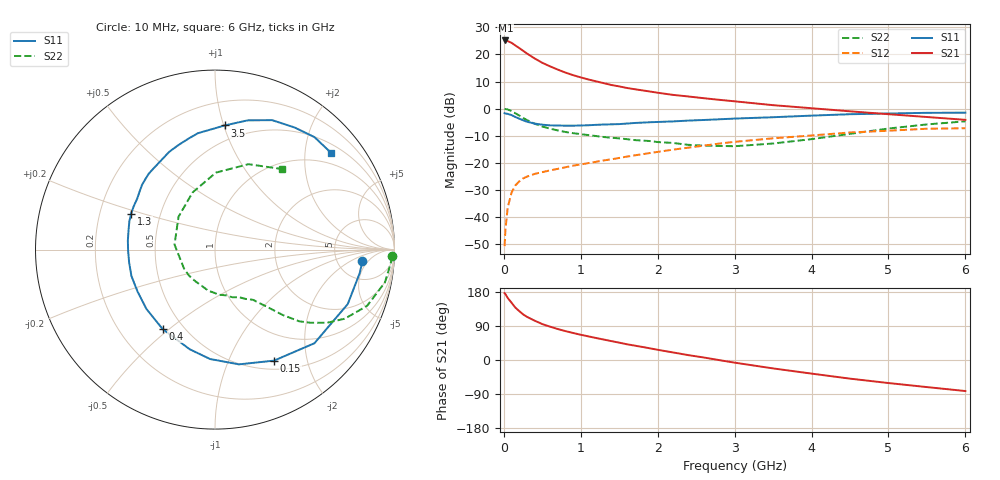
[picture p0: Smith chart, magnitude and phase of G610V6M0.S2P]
! SIEMENS Small Signal Semiconductors
! BFG193
! Si NPN RF Bipolar Junction Transistor in SOT223
! VCE = 10 V  IC = 6 mA
! Common Emitter S-Parameters:  August  1996
# GHz  S  MA  R  50
!  f  S11  S21  S12  S22
! GHz  MAG  ANG  MAG  ANG  MAG  ANG  MAG  ANG
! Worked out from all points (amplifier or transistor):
!   36 points, 10 MHz to 6 GHz, reference 50 ohm
!   highest |S21| = 25.2 dB at 20 MHz (marker M1)
!   |S21| within 3 dB of that: start of sweep to 210.2 MHz
!   unconditionally stable (mu >= 1): 1.089 GHz to 2.532 GHz
!   at 250 MHz: K = 0.37, MSG = 23.6 dB, |S12| = -25.8 dB
!   at 1.4 GHz: K = 1.08, MAG = 12.0 dB, |S12| = -18.7 dB
!   at 6 GHz: K = 0.85, MSG = 1.6 dB, |S12| = -7.2 dB
!   S11 on the Smith chart (normalised r, x): 10 MHz: 8.84, -3.63; 150 MHz: 0.61, -1.49; 400 MHz: 0.39, -0.47; 1.3 GHz: 0.34, +0.18; 3.5 GHz: 0.38, +1.01; 6 GHz: 0.70, +2.59
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0.01  0.8238 -4.6  18.09 176.3  0.0029 84.9  0.9878 -2.2
0.02  0.8169 -9.2  18.09 174.1  0.0057 82.5  0.982 -4.4
0.05  0.7994 -22.3  17.59 163.8  0.0149 78.3  0.9644 -10.9
0.1  0.7609 -43.3  16.38 151.2  0.0282 69.6  0.9034 -20.3
0.15  0.7006 -62.0  14.6 138.2  0.0383 60.4  0.8195 -28.0
0.2  0.6532 -78.2  13.12 129.1  0.0454 55.6  0.7461 -33.1
0.25  0.6102 -92.6  11.68 120.5  0.0515 50.8  0.6712 -37.4
0.3  0.5728 -104.3  10.4 113.9  0.0556 48.0  0.6165 -40.4
0.4  0.5298 -123.5  8.437 103.8  0.0624 44.5  0.5267 -43.9
0.5  0.5054 -139.1  7.001 94.8  0.0674 42.5  0.4676 -46.1
0.6  0.4908 -151.5  6.022 88.0  0.0725 42.6  0.4272 -47.9
0.7  0.4883 -162.4  5.253 81.8  0.0774 42.3  0.3963 -49.7
0.9  0.4841 -179.0  4.144 71.3  0.0887 42.4  0.3526 -52.7
1.1  0.4933 167.7  3.445 62.3  0.099 42.8  0.3248 -57.9
1.3  0.5087 156.8  2.946 53.9  0.1109 42.7  0.2991 -62.7
1.6  0.5302 142.4  2.403 41.5  0.1303 40.9  0.2732 -73.0
2.2  0.5812 120.9  1.792 19.9  0.1752 34.7  0.2326 -99.0
2.8  0.6354 103.5  1.454 -0.3  0.2264 25.1  0.205 -135.1
3.5  0.6936 85.6  1.158 -22.2  0.2831 10.4  0.2272 172.9
4.5  0.7883 66.2  0.892 -49.2  0.3626 -9.7  0.3423 111.3
5.5  0.8366 48.5  0.7 -71.5  0.4255 -35.3  0.5111 68.6
6  0.8418 39.9  0.621 -81.9  0.4346 -50.1  0.5829 50.4
